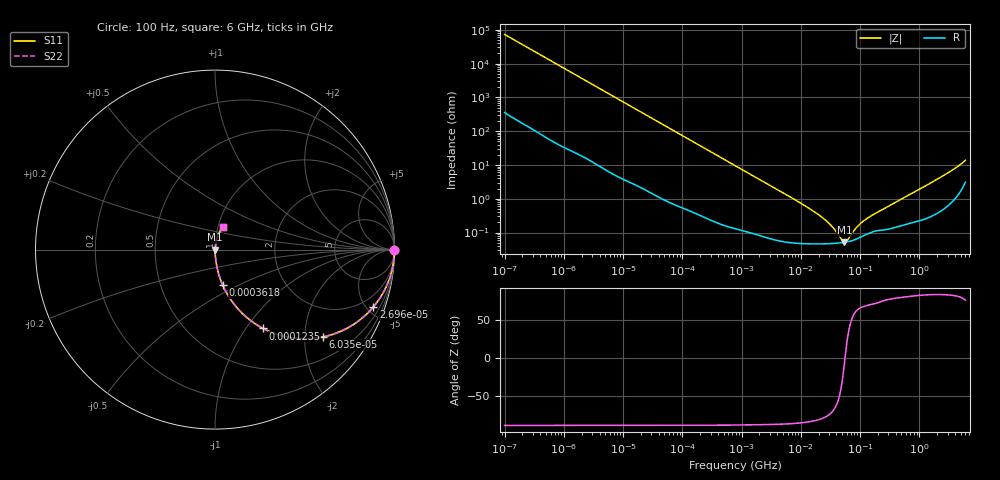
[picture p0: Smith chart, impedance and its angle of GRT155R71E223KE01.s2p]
!Murata Part Number: GRT155R71E223KE01
!These Parameters are Measured in Series Mode Connection
!Data Generated on Jun 19, 2026
!  o--ll--o
!Port1  Port2
!  o------o
!Operation Temp=25[degC], DC Bias Voltage=0[V]
!Freq. Start=100[Hz] Stop=6[GHz] 401[Steps]
# Hz S RI R 50
!Freq.(Hz) S11(Real) S11(Imag) S21(Real) S21(Imag) S12(Real) S12(Imag) S22(Real) S22(Imag)
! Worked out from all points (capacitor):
!   401 points, 100 Hz to 6 GHz, reference 50 ohm
!   read as one part in series: C = 21.8 nF near 109 Hz
!   lowest |Z| = 51.8 mohm at 54.5 MHz (marker M1)
!   series resonance near 55.74 MHz, so ESL is about 370 pH
!   S11 on the Smith chart (normalised r, x): 100 Hz: open; 26.96 kHz: 1.03, -5.49; 60.35 kHz: 1.02, -2.46; 123.5 kHz: 1.01, -1.21; 361.8 kHz: 1.00, -0.41; 6 GHz: 1.06, +0.27
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100  1 -0.00137  8.6e-06 0.00137  8.6e-06 0.00137  1 -0.00137
2008  0.9991 -0.0273  0.000885 0.0273  0.000885 0.0273  0.9991 -0.0273
8801  0.9854 -0.1175  0.0146 0.1175  0.0146 0.1175  0.9854 -0.1175
26957  0.8815 -0.3203  0.1185 0.3203  0.1185 0.3203  0.8815 -0.3203
40335  0.7703 -0.4177  0.2297 0.4177  0.2297 0.4177  0.7703 -0.4177
60352  0.6014 -0.4865  0.3986 0.4865  0.3986 0.4865  0.6014 -0.4865
123542  0.2679 -0.4391  0.7321 0.4391  0.7321 0.4391  0.2679 -0.4391
202169  0.122 -0.323  0.878 0.323  0.878 0.323  0.122 -0.323
361830  0.0428 -0.1975  0.9572 0.1975  0.9572 0.1975  0.0428 -0.1975
774597  0.0106 -0.0958  0.9894 0.0958  0.9894 0.0958  0.0106 -0.0958
2481164  0.00165 -0.0304  0.9983 0.0304  0.9983 0.0304  0.00165 -0.0304
1.555665e7  0.000481 -0.00451  0.9995 0.00451  0.9995 0.00451  0.000481 -0.00451
2.911731e7  0.00047 -0.0019  0.9995 0.0019  0.9995 0.0019  0.00047 -0.0019
3.64232e7  0.000478 -0.0012  0.9995 0.0012  0.9995 0.0012  0.000478 -0.0012
4.983056e7  0.000502 -0.000306  0.9995 0.000306  0.9995 0.000306  0.000502 -0.000306
5.449875e7  0.000514 -6.06e-05  0.9995 6.06e-05  0.9995 6.06e-05  0.000514 -6.06e-05
6.233367e7  0.000536 0.000307  0.9995 -0.000307  0.9995 -0.000307  0.000536 0.000307
8.527865e7  0.000633 0.00119  0.9994 -0.00119  0.9994 -0.00119  0.000633 0.00119
1.115611e8  0.0008 0.00197  0.9992 -0.00197  0.9992 -0.00197  0.0008 0.00197
3.124326e8  0.00131 0.00609  0.9987 -0.00609  0.9987 -0.00609  0.00131 0.00609
2.240541e9  0.00589 0.0417  0.9941 -0.0417  0.9941 -0.0417  0.00589 0.0417
6e9  0.0461 0.1235  0.9539 -0.1235  0.9539 -0.1235  0.0461 0.1235
